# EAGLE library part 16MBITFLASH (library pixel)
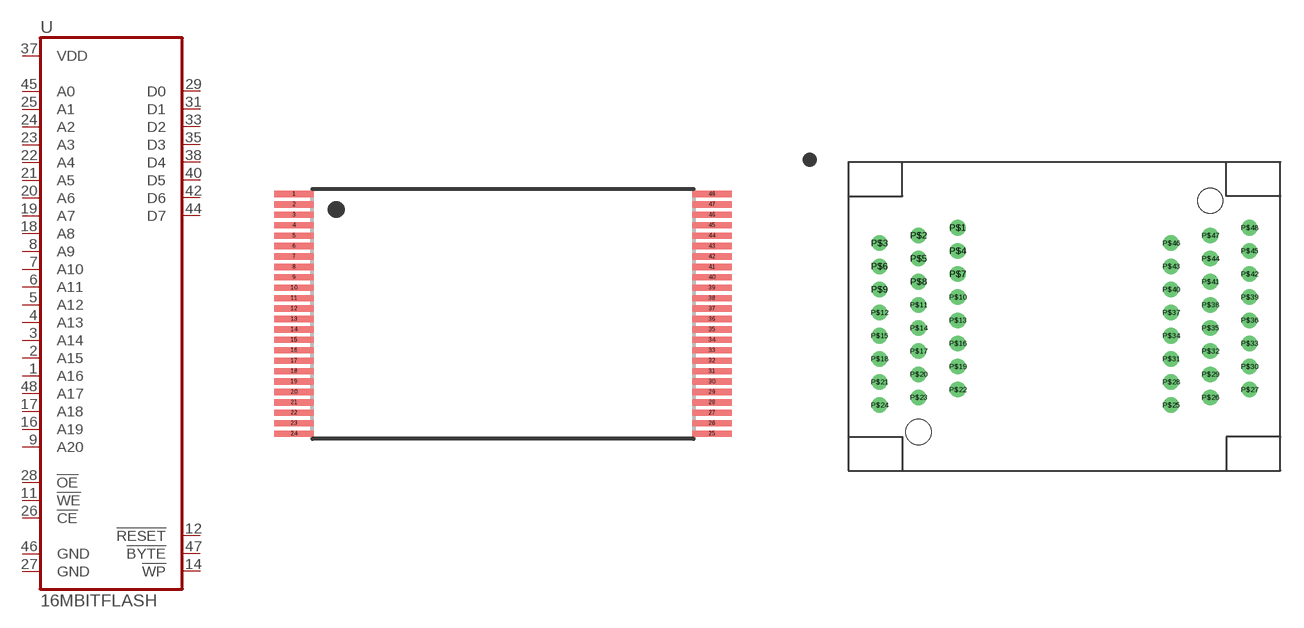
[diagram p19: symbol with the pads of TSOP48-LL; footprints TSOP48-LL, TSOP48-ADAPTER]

Designator prefix -

## 16MBITFLASHLONGLEAD  [TSOP48-LL]
1  A16  in
2  A15  in
3  A14  in
4  A13  in
5  A12  in
6  A11  in
7  A10  in
8  A9  in
9  A20
11  !WE  in
12  !RESET
14  !WP
16  A19
17  A18  in
18  A8  in
19  A7  in
20  A6  in
21  A5  in
22  A4  in
23  A3  in
24  A2  in
25  A1  in
26  !CE  in
27  GND  pwr
28  !OE  in
29  D0
31  D1
33  D2
35  D3
37  VDD  pwr
38  D4
40  D5
42  D6
44  D7
45  A0  in
46  GND  pwr
47  !BYTE
48  A17  in

## 16MBITFLASHSOCKET  [TSOP48-ADAPTER]
P$1  A16  in
P$2  A15  in
P$3  A14  in
P$4  A13  in
P$5  A12  in
P$6  A11  in
P$7  A10  in
P$8  A9  in
P$9  A20
P$11  !WE  in
P$12  !RESET
P$14  !WP
P$16  A19
P$17  A18  in
P$18  A8  in
P$19  A7  in
P$20  A6  in
P$21  A5  in
P$22  A4  in
P$23  A3  in
P$24  A2  in
P$25  A1  in
P$26  !CE  in
P$27  GND  pwr
P$28  !OE  in
P$29  D0
P$31  D1
P$33  D2
P$35  D3
P$37  VDD  pwr
P$38  D4
P$40  D5
P$42  D6
P$44  D7
P$45  A0  in
P$46  GND  pwr
P$47  !BYTE
P$48  A17  in

## 16MBITFLASH  [TSOP48]
1  A16  in
2  A15  in
3  A14  in
4  A13  in
5  A12  in
6  A11  in
7  A10  in
8  A9  in
9  A20
11  !WE  in
12  !RESET
14  !WP
16  A19
17  A18  in
18  A8  in
19  A7  in
20  A6  in
21  A5  in
22  A4  in
23  A3  in
24  A2  in
25  A1  in
26  !CE  in
27  GND  pwr
28  !OE  in
29  D0
31  D1
33  D2
35  D3
37  VDD  pwr
38  D4
40  D5
42  D6
44  D7
45  A0  in
46  GND  pwr
47  !BYTE
48  A17  in

## Footprint TSOP48-LL (pad centres in mm)
48-Lead Thin Small Outline Package (TSOP) 12mm x 20mm SST Package Code: EK Source: http://www.sst.com/dotAsset/40687.pdf
smd 1.9 x 0.3: 1 -10.025,5.75; 2 -10.025,5.25; 3 -10.025,4.75; 4 -10.025,4.25; 5 -10.025,3.75; 6 -10.025,3.25; 7 -10.025,2.75; 8 -10.025,2.25; 9 -10.025,1.75; 10 -10.025,1.25; 11 -10.025,0.75; 12 -10.025,0.25; 13 -10.025,-0.25; 14 -10.025,-0.75; 15 -10.025,-1.25; 16 -10.025,-1.75; 17 -10.025,-2.25; 18 -10.025,-2.75; 19 -10.025,-3.25; 20 -10.025,-3.75; 21 -10.025,-4.25; 22 -10.025,-4.75; 23 -10.025,-5.25; 24 -10.025,-5.75; 25 10.025,-5.75; 26 10.025,-5.25; 27 10.025,-4.75; 28 10.025,-4.25; 29 10.025,-3.75; 30 10.025,-3.25; 31 10.025,-2.75; 32 10.025,-2.25; 33 10.025,-1.75; 34 10.025,-1.25; 35 10.025,-0.75; 36 10.025,-0.25; 37 10.025,0.25; 38 10.025,0.75; 39 10.025,1.25; 40 10.025,1.75; 41 10.025,2.25; 42 10.025,2.75; 43 10.025,3.25; 44 10.025,3.75; 45 10.025,4.25; 46 10.025,4.75; 47 10.025,5.25; 48 10.025,5.75

## Footprint TSOP48-ADAPTER (pad centres in mm)
drill 0.5 pad 0.754: P$1 -6.915,5.75; P$2 -9.455,5.25; P$3 -11.995,4.75; P$4 -6.915,4.25; P$5 -9.455,3.75; P$6 -11.995,3.25; P$7 -6.915,2.75; P$8 -9.455,2.25; P$9 -11.995,1.75; P$10 -6.915,1.25; P$11 -9.455,0.75; P$12 -11.995,0.25; P$13 -6.915,-0.25; P$14 -9.455,-0.75; P$15 -11.995,-1.25; P$16 -6.915,-1.75; P$17 -9.455,-2.25; P$18 -11.995,-2.75; P$19 -6.915,-3.25; P$20 -9.455,-3.75; P$21 -11.995,-4.25; P$22 -6.915,-4.75; P$23 -9.455,-5.25; P$24 -11.995,-5.75; P$25 6.915,-5.75; P$26 9.455,-5.25; P$27 11.995,-4.75; P$28 6.915,-4.25; P$29 9.455,-3.75; P$30 11.995,-3.25; P$31 6.915,-2.75; P$32 9.455,-2.25; P$33 11.995,-1.75; P$34 6.915,-1.25; P$35 9.455,-0.75; P$36 11.995,-0.25; P$37 6.915,0.25; P$38 9.455,0.75; P$39 11.995,1.25; P$40 6.915,1.75; P$41 9.455,2.25; P$42 11.995,2.75; P$43 6.915,3.25; P$44 9.455,3.75; P$45 11.995,4.25; P$46 6.915,4.75; P$47 9.455,5.25; P$48 11.995,5.75
hole 1.65 at 9.455,7.5
hole 1.65 at -9.455,-7.5

## Footprint TSOP48 (pad centres in mm)
48-Pin TSOP OCPL Type 1 (WC Package Code) Source: http://download.micron.com/pdf/datasheets/flash/nand/4gb_nand_m40a.pdf
smd 0.9 x 0.3: 1 -9.75,5.75; 2 -9.75,5.25; 3 -9.75,4.75; 4 -9.75,4.25; 5 -9.75,3.75; 6 -9.75,3.25; 7 -9.75,2.75; 8 -9.75,2.25; 9 -9.75,1.75; 10 -9.75,1.25; 11 -9.75,0.75; 12 -9.75,0.25; 13 -9.75,-0.25; 14 -9.75,-0.75; 15 -9.75,-1.25; 16 -9.75,-1.75; 17 -9.75,-2.25; 18 -9.75,-2.75; 19 -9.75,-3.25; 20 -9.75,-3.75; 21 -9.75,-4.25; 22 -9.75,-4.75; 23 -9.75,-5.25; 24 -9.75,-5.75; 25 9.75,-5.75; 26 9.75,-5.25; 27 9.75,-4.75; 28 9.75,-4.25; 29 9.75,-3.75; 30 9.75,-3.25; 31 9.75,-2.75; 32 9.75,-2.25; 33 9.75,-1.75; 34 9.75,-1.25; 35 9.75,-0.75; 36 9.75,-0.25; 37 9.75,0.25; 38 9.75,0.75; 39 9.75,1.25; 40 9.75,1.75; 41 9.75,2.25; 42 9.75,2.75; 43 9.75,3.25; 44 9.75,3.75; 45 9.75,4.25; 46 9.75,4.75; 47 9.75,5.25; 48 9.75,5.75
